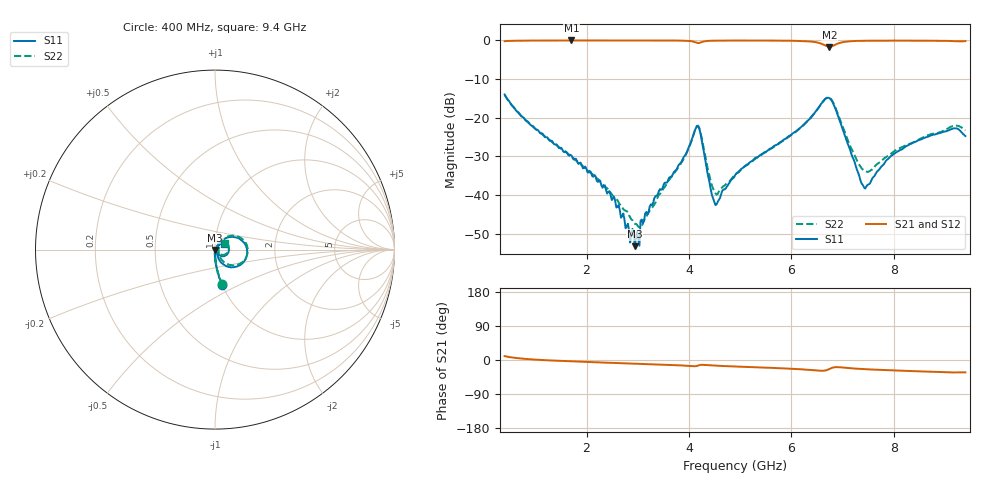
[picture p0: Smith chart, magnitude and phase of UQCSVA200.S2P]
!  Part Number  UQCSVA200  Mounting Orientation: Horizontal
!  Description: Ultra Low ESR Microwave capacitors
!  Application: Coupling, Bypass, Tuning, DC Block
!  Filters, Matching
# GHZ S DB R 50
! Freq  |S11|  S11 Ph  |S21|  S21 Ph  |S12|  S12 Ph  |S22|  S22 Ph
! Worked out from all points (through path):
!   401 points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, 400 MHz to 9.4 GHz, reference 50 ohm
!   highest |S21| = -0.02 dB at 1.705 GHz (marker M1); lowest = -1.7 dB at 6.745 GHz (marker M2)
!   group delay of S21, straight-line fit = 11.1 ps
!   lowest |S11| = -53.2 dB at 2.943 GHz (marker M3), VSWR 1.00, Z = 50.2 - j0.14 ohm
!   |S11| at or under -10 dB: start of sweep to end of sweep
!   |S22| runs from -48.4 to -14.1 dB; largest |S21 - S12| = 0.0082
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0.4  -13.98 -78.8  -0.21 10.2  -0.27 10.2  -14.11 -78.5
0.85  -20.96 -85.0  -0.06 2.4  -0.11 2.5  -21.15 -85.4
1.705  -29.75 -91.0  -0.02 -3.6  -0.05 -3.4  -30.11 -88.3
1.908  -32.34 -93.8  -0.02 -4.7  -0.05 -4.4  -32.31 -87.3
2.493  -41.29 -87.2  -0.02 -7.5  -0.03 -7.3  -39.74 -77.3
2.808  -47.43 -66.5  -0.02 -9.0  -0.03 -8.8  -44.45 -59.7
2.943  -53.24 -39.7  -0.03 -9.7  -0.03 -9.5  -47.46 -50.7
2.988  -49.47 -27.9  -0.03 -9.9  -0.03 -9.7  -47.74 -42.3
3.078  -46.34 9.7  -0.03 -10.3  -0.03 -10.1  -48.05 23.1
3.415  -38.90 50.9  -0.03 -11.8  -0.03 -11.7  -39.94 55.9
3.888  -30.44 53.6  -0.08 -14.5  -0.07 -14.4  -30.90 61.8
4.158  -22.22 3.6  -0.65 -15.7  -0.64 -15.5  -22.10 15.0
4.225  -24.06 -36.1  -0.55 -12.9  -0.54 -12.8  -23.77 -23.1
4.495  -41.76 -21.4  -0.08 -14.8  -0.06 -14.8  -39.02 -14.7
4.9  -34.92 53.0  -0.04 -17.2  -0.03 -17.1  -34.84 48.1
6.408  -19.51 41.0  -0.34 -26.6  -0.37 -27.0  -19.57 44.7
6.745  -14.96 -17.4  -1.68 -23.6  -1.73 -23.5  -14.85 -10.6
6.993  -22.56 -65.8  -0.50 -19.7  -0.53 -19.4  -21.94 -55.5
7.42  -38.02 -21.1  -0.11 -24.1  -0.11 -23.9  -33.55 -16.4
7.915  -30.34 48.1  -0.07 -27.0  -0.06 -26.9  -29.60 39.0
9.13  -22.95 40.0  -0.17 -32.7  -0.16 -32.6  -22.27 44.2
9.4  -24.76 30.7  -0.19 -32.6  -0.19 -32.6  -23.29 32.1
